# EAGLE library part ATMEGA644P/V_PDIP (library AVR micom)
ATMEGA644P/V PDIP pacage AVR micon series. producted by ATMEL.Co
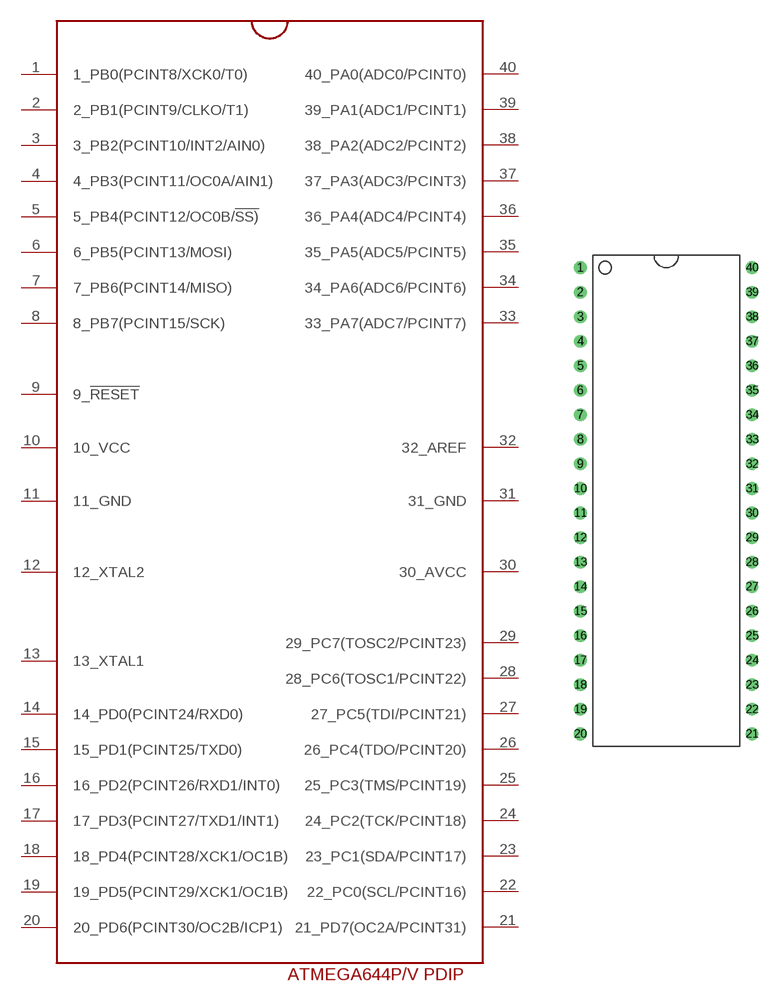
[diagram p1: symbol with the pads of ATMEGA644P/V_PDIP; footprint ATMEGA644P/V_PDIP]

Designator prefix -

## ATMEGA644P/V_PDIP  [ATMEGA644P/V_PDIP]
1  1_PB0(PCINT8/XCK0/T0)
2  2_PB1(PCINT9/CLKO/T1)
3  3_PB2(PCINT10/INT2/AIN0)
4  4_PB3(PCINT11/OC0A/AIN1)
5  5_PB4(PCINT12/OC0B/!SS)
6  6_PB5(PCINT13/MOSI)
7  7_PB6(PCINT14/MISO)
8  8_PB7(PCINT15/SCK)
9  9_!RESET
10  10_VCC
11  11_GND
12  12_XTAL2
13  13_XTAL1
14  14_PD0(PCINT24/RXD0)
15  15_PD1(PCINT25/TXD0)
16  16_PD2(PCINT26/RXD1/INT0)
17  17_PD3(PCINT27/TXD1/INT1)
18  18_PD4(PCINT28/XCK1/OC1B)
19  19_PD5(PCINT29/XCK1/OC1B)
20  20_PD6(PCINT30/OC2B/ICP1)
21  21_PD7(OC2A/PCINT31)
22  22_PC0(SCL/PCINT16)
23  23_PC1(SDA/PCINT17)
24  24_PC2(TCK/PCINT18)
25  25_PC3(TMS/PCINT19)
26  26_PC4(TDO/PCINT20)
27  27_PC5(TDI/PCINT21)
28  28_PC6(TOSC1/PCINT22)
29  29_PC7(TOSC2/PCINT23)
30  30_AVCC
31  31_GND
32  32_AREF
33  33_PA7(ADC7/PCINT7)
34  34_PA6(ADC6/PCINT6)
35  35_PA5(ADC5/PCINT5)
36  36_PA4(ADC4/PCINT4)
37  37_PA3(ADC3/PCINT3)
38  38_PA2(ADC2/PCINT2)
39  39_PA1(ADC1/PCINT1)
40  40_PA0(ADC0/PCINT0)

## Footprint ATMEGA644P/V_PDIP (pad centres in mm)
ATMEGA644P/V 10AU/20AU 40pin(PDIP) pacage AVR micon series. producted by ATMEL.Co
drill 0.8: 1 -8.89,22.86; 2 -8.89,20.32; 3 -8.89,17.78; 4 -8.89,15.24; 5 -8.89,12.7; 6 -8.89,10.16; 7 -8.89,7.62; 8 -8.89,5.08; 9 -8.89,2.54; 10 -8.89,0; 11 -8.89,-2.54; 12 -8.89,-5.08; 13 -8.89,-7.62; 14 -8.89,-10.16; 15 -8.89,-12.7; 16 -8.89,-15.24; 17 -8.89,-17.78; 18 -8.89,-20.32; 19 -8.89,-22.86; 20 -8.89,-25.4; 21 8.89,-25.4; 22 8.89,-22.86; 23 8.89,-20.32; 24 8.89,-17.78; 25 8.89,-15.24; 26 8.89,-12.7; 27 8.89,-10.16; 28 8.89,-7.62; 29 8.89,-5.08; 30 8.89,-2.54; 31 8.89,0; 32 8.89,2.54; 33 8.89,5.08; 34 8.89,7.62; 35 8.89,10.16; 36 8.89,12.7; 37 8.89,15.24; 38 8.89,17.78; 39 8.89,20.32; 40 8.89,22.86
